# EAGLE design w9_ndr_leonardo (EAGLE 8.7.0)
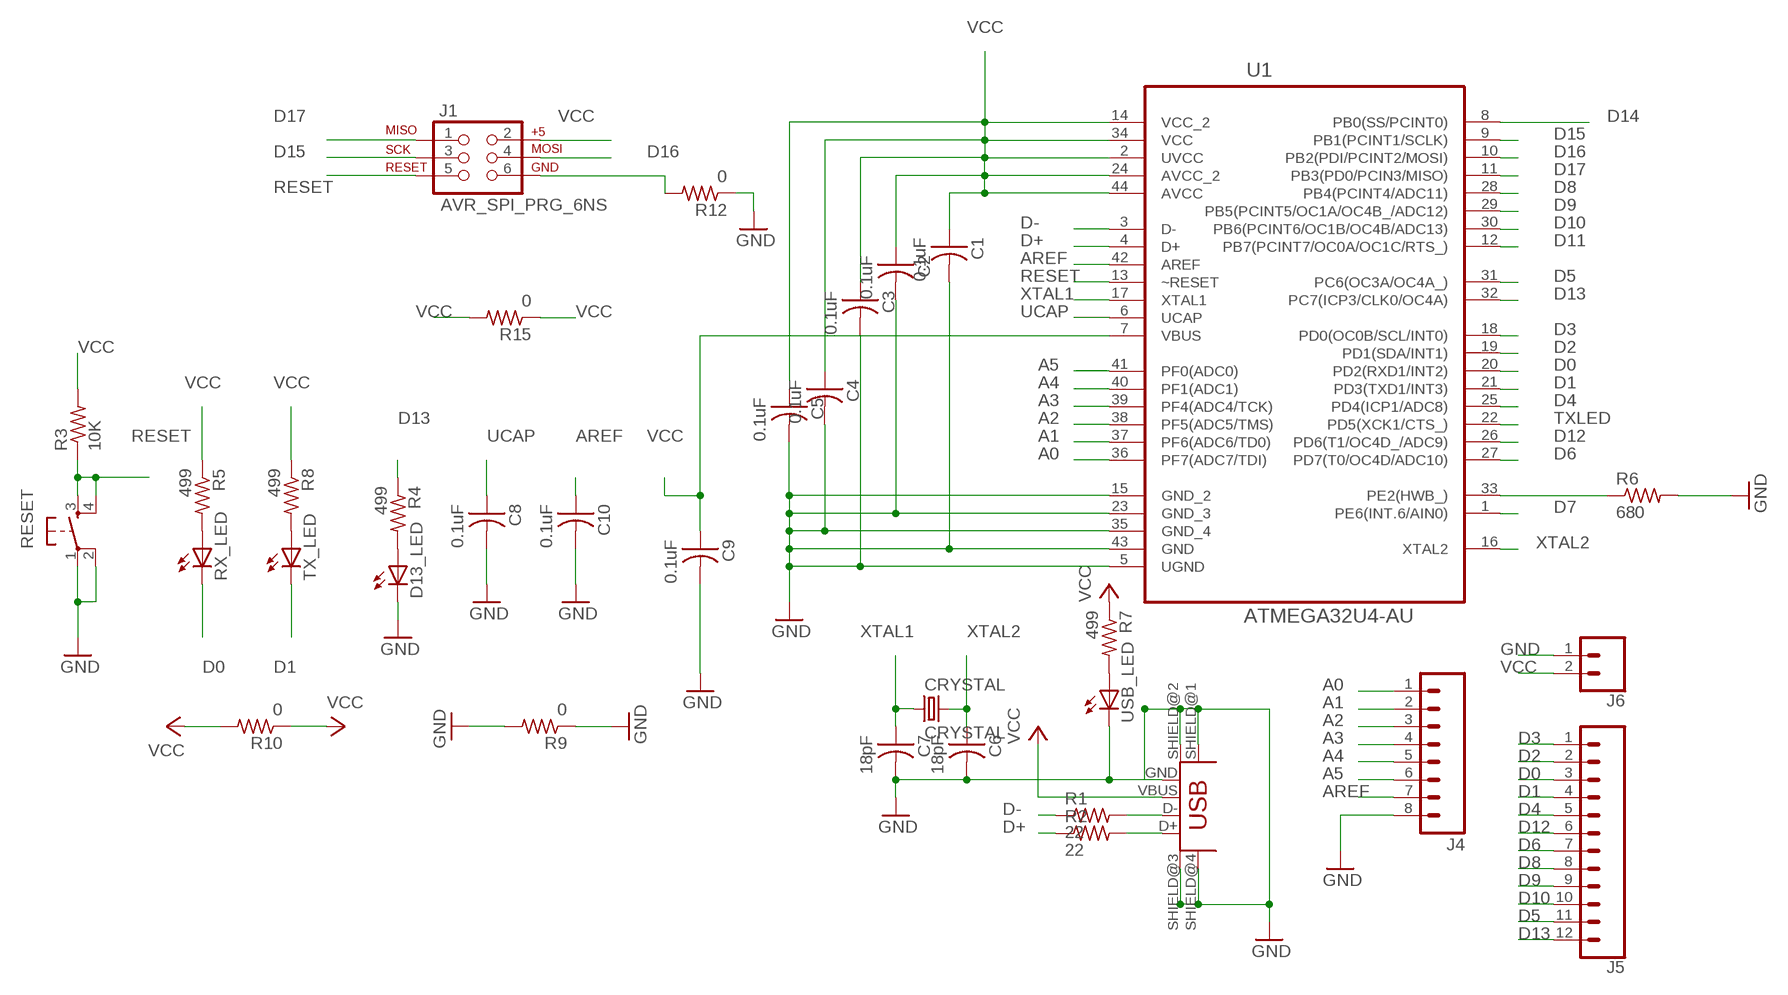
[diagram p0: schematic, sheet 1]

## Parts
C1  0.1uF  CAP-US1206FAB  [C1206FAB]
C2  0.1uF  CAP-US1206FAB  [C1206FAB]
C3  0.1uF  CAP-US1206FAB  [C1206FAB]
C4  0.1uF  CAP-US1206FAB  [C1206FAB]
C5  0.1uF  CAP-US1206FAB  [C1206FAB]
C6  18pF  CAP-US1206FAB  [C1206FAB]
C7  18pF  CAP-US1206FAB  [C1206FAB]
C8  0.1uF  CAP-US1206FAB  [C1206FAB]
C9  0.1uF  CAP-US1206FAB  [C1206FAB]
C10  0.1uF  CAP-US1206FAB  [C1206FAB]
CRYSTAL  CRYSTAL  [2-SMD-5X3MM]
D13_LED  LED1206  [1206]
J1  AVR_SPI_PRG_6NS  [2X3-NS]
J4  M08NO_SILK  [1X08_PIN1_NO_SILK]
J5  CONN_12NO_SILK  [1X12_NO_SILK]
J6  CONN_021X02_NO_SILK  [1X02_NO_SILK]
R1  22  RES-US1206FAB  [R1206FAB]
R2  22  RES-US1206FAB  [R1206FAB]
R3  10K  RES-US1206FAB  [R1206FAB]
R4  499  RESISTOR1206  [1206]
R5  499  RESISTOR1206  [1206]
R6  680  RES-US1206FAB  [R1206FAB]
R7  499  RESISTOR1206  [1206]
R8  499  RESISTOR1206  [1206]
R9  0  RES-US1206FAB  [R1206FAB]
R10  0  RES-US1206FAB  [R1206FAB]
R12  0  RES-US1206FAB  [R1206FAB]
R15  0  RES-US1206FAB  [R1206FAB]
RESET  6MM_SWITCH6MM_SWITCH  [6MM_SWITCH]
RX_LED  LED1206  [1206]
TX_LED  LED1206  [1206]
U1  ATMEGA32U4-AU  [QFP80P1200X1200X120-44N]
USB_LED  LED1206  [1206]
USB_UPLOAD  USB_MINIB  [USB_MINIB]

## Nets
A0: J4.1 U1.36(PF7(ADC7/TDI))
A1: J4.2 U1.37(PF6(ADC6/TD0))
A2: J4.3 U1.38(PF5(ADC5/TMS))
A3: J4.4 U1.39(PF4(ADC4/TCK))
A4: J4.5 U1.40(PF1(ADC1))
A5: J4.6 U1.41(PF0(ADC0))
AREF: C10.1 J4.7 U1.42(AREF)
D0: J5.3 RX_LED.2(C) U1.20(PD2(RXD1/INT2))
D1: J5.4 TX_LED.2(C) U1.21(PD3(TXD1/INT3))
D2: J5.2 U1.19(PD1(SDA/INT1))
D3: J5.1 U1.18(PD0(OC0B/SCL/INT0))
D4: J5.5 U1.25(PD4(ICP1/ADC8))
D5: J5.11 U1.31(PC6(OC3A/OC4A_))
D6: J5.7 U1.27(PD7(T0/OC4D/ADC10))
D7: U1.1(PE6(INT.6/AIN0))
D8: J5.8 U1.28(PB4(PCINT4/ADC11))
D9: J5.9 U1.29(PB5(PCINT5/OC1A/OC4B_/ADC12))
D10: J5.10 U1.30(PB6(PCINT6/OC1B/OC4B/ADC13))
D11: U1.12(PB7(PCINT7/OC0A/OC1C/RTS_))
D12: J5.6 U1.26(PD6(T1/OC4D_/ADC9))
D13: J5.12 R4.1 U1.32(PC7(ICP3/CLK0/OC4A))
D14: U1.8(PB0(SS/PCINT0))
D15: J1.3 U1.9(PB1(PCINT1/SCLK))
D16: J1.4 U1.10(PB2(PDI/PCINT2/MOSI))
D17: J1.1 U1.11(PB3(PD0/PCIN3/MISO))
D+: R2.1 U1.4(D+)
D-: R1.1 U1.3(D-)
GND: C1.2 C2.2 C3.2 C4.2 C5.2 C6.2 C7.2 C8.2 C9.2 C10.2 D13_LED.2(C) J4.8 J6.1 R6.2 R9.1 R9.2 R12.1 RESET.1(P) RESET.2(P1) U1.5(UGND) U1.15(GND_2) U1.23(GND_3) U1.35(GND_4) U1.43(GND) USB_LED.2(C) USB_UPLOAD.GND USB_UPLOAD.SHIELD@1(SHIELD) USB_UPLOAD.SHIELD@2(SHIELD1) USB_UPLOAD.SHIELD@3(SHIELD2) USB_UPLOAD.SHIELD@4(SHIELD3)
N$1: R1.2 USB_UPLOAD.D-
N$2: R2.2 USB_UPLOAD.D+
N$3: D13_LED.1(A) R4.2
N$4: R5.2 RX_LED.1(A)
N$5: R7.2 USB_LED.1(A)
N$6: R8.2 TX_LED.1(A)
N$13: J1.6 R12.2
N$35: R6.1 U1.33(PE2(HWB_))
RESET: J1.5 R3.1 RESET.3(S) RESET.4(S1) U1.13(~RESET)
TXLED: U1.22(PD5(XCK1/CTS_))
UCAP: C8.1 U1.6(UCAP)
VCC: C1.1 C2.1 C3.1 C4.1 C5.1 C9.1 J1.2 J6.2 R3.2 R5.1 R7.1 R8.1 R10.1 R10.2 R15.1 R15.2 U1.2(UVCC) U1.7(VBUS) U1.14(VCC_2) U1.24(AVCC_2) U1.34(VCC) U1.44(AVCC) USB_UPLOAD.VBUS
XTAL1: C7.1 CRYSTAL.P$1 U1.17(XTAL1)
XTAL2: C6.1 CRYSTAL.P$2 U1.16(XTAL2)

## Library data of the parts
C1-C10 = fab:CAP-US
CRYSTAL = fab:CRYSTAL
D13_LED RX_LED TX_LED USB_LED = ng:LED
J1 = SparkFun-ConnectorsModified:AVR_SPI_PRG_6: AVR ISP 6 Pin This is the reduced ISP connector for AVR programming. Common on Arduino. This footprint will take up less PCB space and can be used with a 10-pin to 6-pin adapter such as SKU: BOB-08508 **Special note about "TEST_POINT" package. The stop mask is on the top side, so if you want your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
J4 = SparkFun-ConnectorsModified:M08: Header 8 Standard 8-pin 0.1" header. Use with straight break away headers (SKU : PRT-00116), right angle break away headers (PRT-00553), swiss pins (PRT-00743), machine pins (PRT-00117), and female headers (PRT-00115).
J5 = SparkFun-Connectors:CONN_12: Multi connection point. Often used as Generic Header-pin footprint for 0.1 inch spaced/style header connections On any of the 0.1 inch spaced packages, you can populate with these: Break Away Headers - Straight (PRT-00116) Break Away Male Headers - Right Angle (PRT-00553) Female Headers (PRT-00115)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
J6 = SparkFun-Connectors:CONN_02: Multi connection point. Often used as Generic Header-pin footprint for 0.1 inch spaced/style header connections
R1-R3 R6 R9 R10 R12 R15 = fab:RES-US: Resistor (US Symbol)
R4 R5 R7 R8 = ng:RESISTOR
RESET = fab:6MM_SWITCH: OMRON SWITCH
U1 = Atmel_By_element14_Batch_1:ATMEGA32U4-AU: 8-bit Microcontroller with ISP Flash and USB Controller; MPN: ATMEGA32U4-AU; OC_FARNELL: 1748525; OC_NEWARK: 26R5633; PACKAGE: TQFP-44; SUPPLIER: Atmel
USB_UPLOAD = fab:USB_MINIB

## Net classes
0 default: width 0.305 mm, drill 0.305 mm, clearance 0.305 mm

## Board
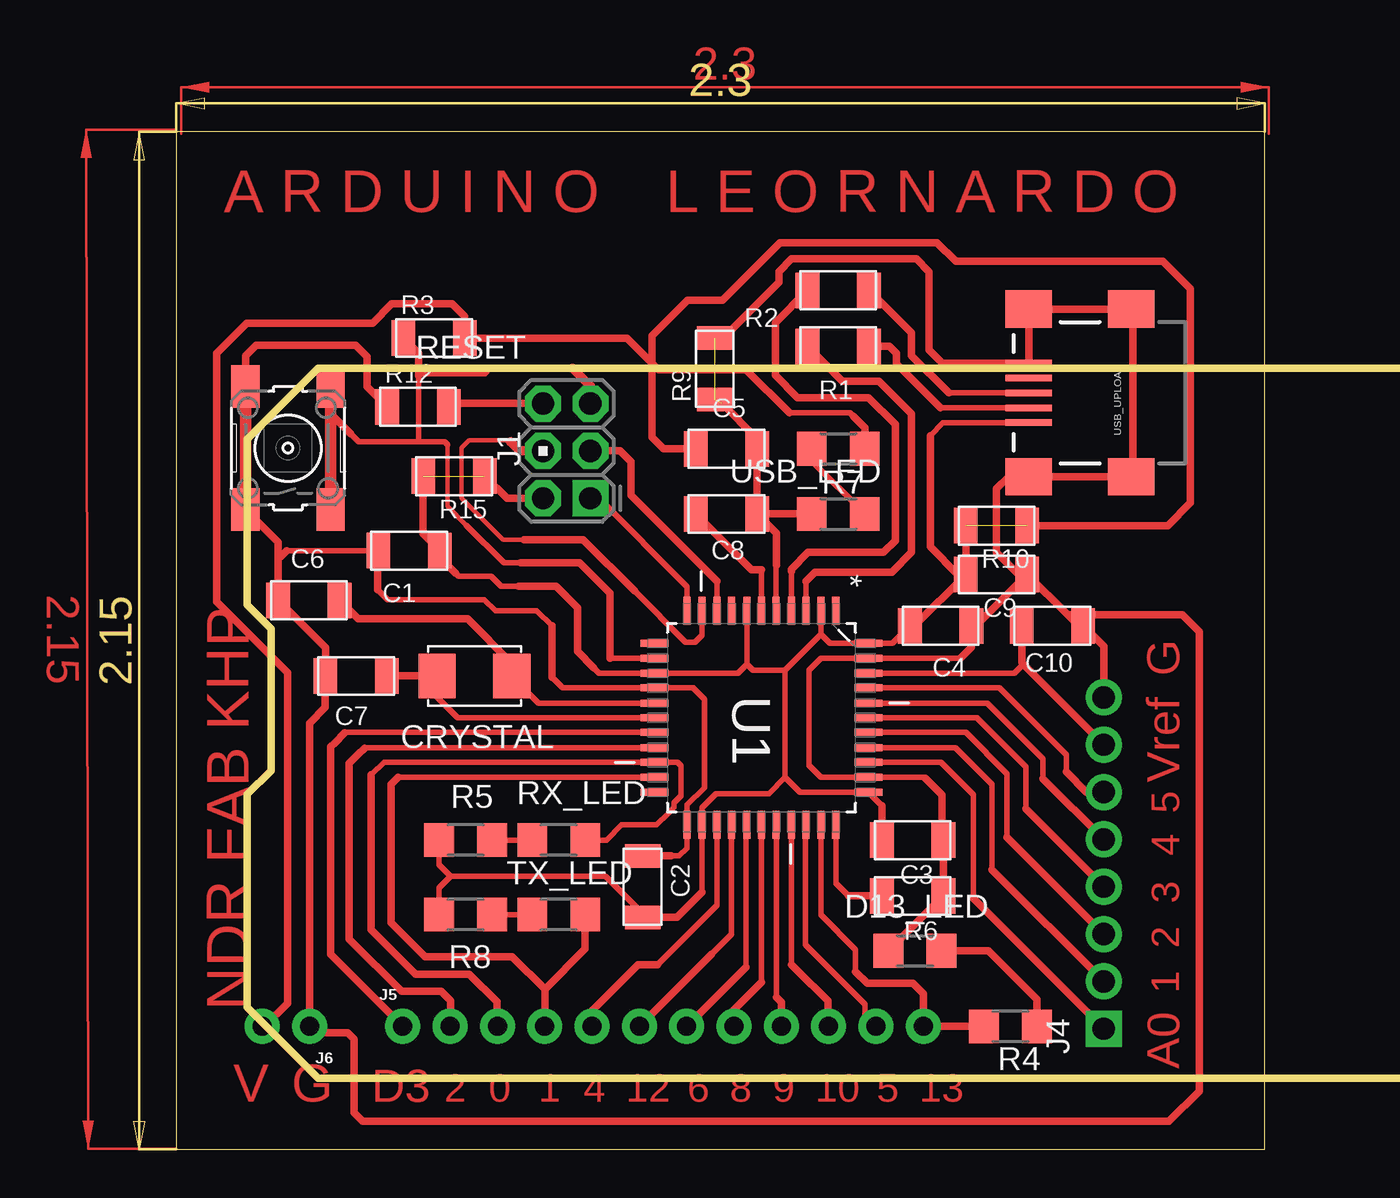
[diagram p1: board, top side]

Size 60.72 x 56.42 mm. Coordinates in mm from the lower left corner, seen from the top.
Outline: 2.3,0 60.72,0 60.72,54.61 2.3,54.61 2.3,0
Copper layers (1*16): Top 0.035mm / dielectric 1.5mm / Bottom 0.035mm
Design rules "default *": minimum track width 10mil, minimum drill 24mil, track to track 0.4mm, track to pad 0.4mm, pad to pad 0.4mm, via to via 0.4mm, smd to smd 0.4mm, copper to edge 40mil, drill to drill 0.4mm, minimum pad ring 10mil, minimum via ring 8mil, stop-mask expansion 4mil, vias tented up to drill 0mil, thermal gap 10mil
Milling: area 6.1,3.8 to 106.4,41.9

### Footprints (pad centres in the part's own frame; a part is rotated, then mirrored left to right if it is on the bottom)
C1206FAB = smd 1.27 x 1.905: 1 -1.651,0; 2 1.651,0
2-SMD-5X3MM = smd 2 x 2.4: P$1 -2,0; P$2 2,0
1206 = smd 1.6 x 1.803: 1 -1.422,0; 2 1.422,0
2X3-NS = drill 1.2 pad 1.93 square: 1 -2.54,-1.27 | drill 1.2 pad 1.93 octagon: 2 -2.54,1.27; 3 0,-1.27; 4 0,1.27; 5 2.54,-1.27; 6 2.54,1.27
1X08_PIN1_NO_SILK = drill 1.2 pad 1.93 square: 1 0,0 | drill 1.2 pad 1.93: 2 2.54,0; 3 5.08,0; 4 7.62,0; 5 10.16,0; 6 12.7,0; 7 15.24,0; 8 17.78,0
1X12_NO_SILK = drill 1.016 pad 1.88: 1 0,0; 2 2.54,0; 3 5.08,0; 4 7.62,0; 5 10.16,0; 6 12.7,0; 7 15.24,0; 8 17.78,0; 9 20.32,0; 10 22.86,0; 11 25.4,0; 12 27.94,0
1X02_NO_SILK = drill 1.016 pad 1.88: 1 0,0; 2 2.54,0
R1206FAB = smd 1.27 x 1.905: 1 -1.651,0; 2 1.651,0
6MM_SWITCH = smd 2.286 x 1.524: 1 -3.302,2.286; 2 3.302,2.286; 3 -3.302,-2.286; 4 3.302,-2.286
QFP80P1200X1200X120-44N = smd 1.5 x 0.38: 1 -5.74,3.988; 2 -5.74,3.2; 3 -5.74,2.388; 4 -5.74,1.6; 5 -5.74,0.787; 6 -5.74,0; 7 -5.74,-0.787; 8 -5.74,-1.6; 9 -5.74,-2.388; 10 -5.74,-3.2; 11 -5.74,-3.988; 23 5.74,-3.988; 24 5.74,-3.2; 25 5.74,-2.388; 26 5.74,-1.6; 27 5.74,-0.787; 28 5.74,0; 29 5.74,0.787; 30 5.74,1.6; 31 5.74,2.388; 32 5.74,3.2; 33 5.74,3.988 | smd 0.38 x 1.5: 12 -3.988,-5.74; 13 -3.2,-5.74; 14 -2.388,-5.74; 15 -1.6,-5.74; 16 -0.787,-5.74; 17 0,-5.74; 18 0.787,-5.74; 19 1.6,-5.74; 20 2.388,-5.74; 21 3.2,-5.74; 22 3.988,-5.74; 34 3.988,5.74; 35 3.2,5.74; 36 2.388,5.74; 37 1.6,5.74; 38 0.787,5.74; 39 0,5.74; 40 -0.787,5.74; 41 -1.6,5.74; 42 -2.388,5.74; 43 -3.2,5.74; 44 -3.988,5.74
USB_MINIB = smd 2.5 x 0.35: D+ 3.77,0; D- 3.77,0.8; GND 3.77,-1.6; ID 3.77,-0.8; VBUS 3.77,1.6 | smd 2.5 x 2: SHIELD@1 -1.73,-4.5; SHIELD@2 -1.73,4.5; SHIELD@3 3.77,4.5; SHIELD@4 3.77,-4.5

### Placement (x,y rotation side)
C1  14.8,32.13 180 top
C2  27.33,14.09 90 top
C3  41.83,16.59 0 top
C4  43.33,28.09 0 top
C5  31.83,37.59 0 top
C6  9.41,29.46 180 top
C7  11.95,25.4 180 top
C8  31.83,34.09 0 top
C9  46.33,30.84 0 top
C10  49.33,28.09 0 top
CRYSTAL  18.3,25.4 0 top
D13_LED  41.96,10.66 180 top
J1  23.26,37.48 90 top
J4  52.08,6.47 90 top
J5  14.46,6.59 0 top
J6  9.46,6.59 180 top
R1  37.83,43.09 0 top
R2  37.83,46.09 0 top
R3  16.13,43.54 0 top
R4  47.08,6.59 0 top
R5  17.83,16.59 0 top
R6  41.83,13.59 0 top
R7  37.83,37.59 180 top
R8  17.83,12.59 0 top
R9  31.2,41.88 90 top
R10  46.33,33.47 180 top
R12  15.27,39.84 0 top
R15  17.21,36.12 180 top
RESET  8.29,37.63 90 top
RX_LED  22.83,16.59 0 top
TX_LED  22.83,12.59 0 top
U1  33.71,23.16 270 top
USB_LED  37.83,34.09 180 top
USB_UPLOAD  51.83,40.59 180 top

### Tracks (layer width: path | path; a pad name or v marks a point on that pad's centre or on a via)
A0
  Top 0.305: U1.36 43.34,20.77 45.08,19.03 45.08,13.47
  Top 0.406: 45.08,13.47 J4.1
A1
  Top 0.305: U1.37 44.12,21.56 46.08,19.59 46.08,15.01
  Top 0.406: 46.08,15.01 J4.2
A2
  Top 0.305: U1.38 44.68,22.37 46.89,20.16 46.89,16.74
  Top 0.406: 46.89,16.74 J4.3
A3
  Top 0.305: U1.39 45.27,23.16 47.89,20.53 47.89,18.28
  Top 0.406: 47.89,18.28 J4.4
A4
  Top 0.305: U1.40 45.85,23.95 48.83,20.97 48.83,19.88
  Top 0.406: 48.83,19.88 J4.5
A5
  Top 0.305: U1.41 46.49,24.76 50.08,21.17 50.08,20.25
  Top 0.406: 50.08,20.25 51.16,19.17 J4.6
AREF
  Top 0.305: U1.42 47.28,25.55 47.76,26.03
  Top 0.406: J4.7 47.76,26.03 47.68,26.11 C10.1
D0
  Top 0.305: 12.77,20.09 13.46,20.78 U1.20 27.98,20.78 29.21,20.78 29.39,20.59 29.39,20.34 29.39,18.97 29.02,18.59 29.02,18.34 28.69,18.02 28.08,17.41 26.21,17.41 25.39,16.59 RX_LED.2
  Top 0.406: 12.77,20.09 12.77,11.78 15.14,9.41 18.02,9.41 19.52,7.91 19.52,6.61 J5.3 19.58,6.59
D1
  Top 0.305: 14.21,19.97 14.22,19.96 U1.21
  Top 0.406: 14.21,19.97 13.83,19.59 13.83,12.16 15.64,10.34 20.33,10.34 22.08,8.59 | 22.08,8.59 J5.4 | TX_LED.2 24.25,10.77 22.08,8.59
D2
  Top 0.305: U1.19 12.42,21.56 12.05,21.19
  Top 0.406: 12.39,21.53 12.05,21.19 11.58,20.72 11.58,11.28 14.39,8.47 16.52,8.47 17.02,7.97 17.02,6.62 J5.2
D3
  Top 0.305: 10.82,21.83 11.36,22.37 U1.18
  Top 0.406: 11.33,22.34 10.82,21.83 10.58,21.59 10.58,10.47 J5.1
D4
  Top 0.305: U1.25 31.33,13.09 28.14,9.91
  Top 0.406: J5.5 24.62,7.44 27.08,9.91 28.14,9.91
D5
  Top 0.305: U1.31 36.08,17.4 36.08,10.97 39.27,7.78 39.27,7.18 J5.11
D6
  Top 0.305: U1.27 32.89,17.39 32.89,9.78
  Top 0.406: J5.7 32.32,9.2 32.89,9.78
D8
  Top 0.305: 33.71,8.97 U1.28
  Top 0.406: 33.71,8.97 32.21,7.47 32.21,6.62 J5.8
D9
  Top 0.305: U1.29 34.52,17.4 34.52,8.16
  Top 0.406: J5.9 34.78,7.9 34.66,8.02 34.52,8.16
D10
  Top 0.305: 35.6,9.64 35.31,9.93 U1.30
  Top 0.406: 35.33,9.91 35.6,9.64 37.27,7.97 37.27,6.64 J5.10
D12
  Top 0.305: U1.26 32.11,11.55 31.03,10.46
  Top 0.406: J5.6 31.03,10.46
D13
  Top 0.305: 38.77,9.53 38.77,10.72 36.91,12.58 U1.32
  Top 0.406: R4.1 J5.12 42.39,8.34 41.83,8.91 39.39,8.91 38.77,9.53
D15
  Top 0.305: U1.9 31.32,30.48
  Top 0.406: J1.3 26.13,37.48 26.71,36.91 26.71,35.09 31.32,30.48
D16
  Top 0.254: 20.96,32.72 19.83,32.72 17.61,34.94 17.61,37.66 18.02,38.06 20.14,38.06 20.24,37.97 20.36,37.84
  Top 0.305: U1.10 30.51,27.59 30.14,27.22 29.64,27.22 26.89,29.97
  Top 0.406: 26.89,29.97 24.14,32.72 20.96,32.72
  Top 0.508: J1.4 20.73,37.48 20.24,37.97
D17
  Top 0.305: U1.11 29.72,30.2 24.98,34.94 J1.1
D+
  Top 0.305: U1.4 35.31,31.01
  Top 0.406: 35.31,31.01 35.31,31.14 36.21,32.03 40.27,32.03 40.89,32.66 40.89,38.91 39.46,40.34 35.64,40.34 34.46,41.53 34.46,44.37 R2.1
D-
  Top 0.305: U1.3 36.1,30.49
  Top 0.406: R1.1 38.05,41.22 40.02,41.22 41.77,39.47 41.77,32.03 40.71,30.97 36.58,30.97 36.1,30.49
GND  (2 unrouted)
  Top 0.305: U1.5 34.5,31.32 34.52,31.34 | 22.46,25.34 23.04,24.76 U1.15 30.06,24.76 30.06,24.74 30.64,24.16 30.64,19.41 29.72,18.49 U1.23 29.71,17.4 29.71,16.16 29.3,15.74 28.86,15.74 | RESET.1 6.52,33.82 | 44.39,26.36 U1.43 36.91,26.36 36.25,25.7 36.25,20.62 36.91,19.96 U1.35 42.47,19.96 42.52,19.91 | C1.2 8.21,32.13 | 22.46,28.09 21.64,28.91 19.43,28.91 18.83,29.5 13.64,29.5 13.11,30.03
  Top 0.406: 42.52,19.91 43.39,19.03 43.39,16.68 C3.2 R6.2 D13_LED.2 | 53.39,36.09 USB_UPLOAD.SHIELD@3 46.99,36.09 46.33,35.44 46.33,32.03 47.75,30.61 | 53.39,36.09 USB_UPLOAD.SHIELD@2 | RESET.2 6.01,42.59 6.57,43.16 11.93,43.16 12.55,42.53 12.55,40.91 R12.1 | C2.2 28.86,15.74 | 34.52,31.34 34.52,33.06 C8.2 | C8.2 USB_LED.2 | C8.2 C5.2 33.48,38.13 31.58,40.03 | 22.46,25.34 22.46,28.09 | J4.8 52.08,27 C10.2 50.73,28.09 50.15,28.68 | 50.15,28.68 C9.2 47.75,30.61 | 47.75,30.61 45.23,28.09 C4.2 44.98,26.95 44.39,26.36 | 9.52,6.53 J6.1 | 53.39,36.09 53.64,36.34 53.64,45.01 USB_UPLOAD.SHIELD@1 USB_UPLOAD.SHIELD@4 USB_UPLOAD.GND 43.42,42.19 42.71,42.91 42.71,47.09 42.02,47.78 35.33,47.78 34.64,47.09 34.64,46.53 31.65,43.53 R9.2 | 13.11,30.03 13.11,32.09 C1.2 | J6.1 9.8,6.25 11.49,6.25 11.85,5.89 11.85,1.95 12.3,1.5 55.58,1.5 57.21,3.12 57.21,27.77 56.3,28.68 50.15,28.68 | 7.76,31.81 C6.2 10.3,26.92 C7.2 10.3,23.72 9.46,22.88 J6.1 | 7.76,31.81 7.76,32.58 6.52,33.82 | 8.21,32.13 7.9,31.81 7.76,31.81
  Top 0.61: RESET.1 RESET.2
N$1
  Top 0.305: USB_UPLOAD.D- 43.32,39.79
  Top 0.406: 43.32,39.79 40.96,42.16 40.96,42.72 40.58,43.09 R1.2
N$2
  Top 0.305: USB_UPLOAD.D+ 43.77,40.59
  Top 0.406: 43.77,40.59 41.77,42.59 41.77,43.81 R2.2
N$3
  Top 0.406: R4.2 48.5,8.05 45.89,10.66 D13_LED.1
N$4
  Top 0.305: R5.2 RX_LED.1
N$5
  Top 0.305: R7.2 36.41,36.94 USB_LED.1
N$6
  Top 0.305: R8.2 TX_LED.1
N$13
  Top 0.406: R12.2 17.11,40.03 21.98,40.03
  Top 0.508: 21.98,40.03 J1.6
N$35
  Top 0.305: U1.33 37.7,14.88 37.7,14.48 37.7,14.29 38.39,13.59
  Top 0.406: 38.39,13.59 R6.1
RESET
  Top 0.254: 17.86,33.5 16.86,34.5 16.86,37.81
  Top 0.305: U1.13 25.6,26.36 25.58,26.34 | 20.77,31.47 19.89,31.47 17.86,33.5 | 16.86,37.81 16.71,37.97 15.3,37.97 | 15.3,37.97 12.08,37.97 11.64,38.41 | 15.3,41.5 15.3,37.97 | 19.14,41.91 18.86,41.62 15.36,41.62 15.3,41.69
  Top 0.406: RESET.4 10.58,39.47 11.64,38.41 | 25.58,26.34 25.58,29.84 23.96,31.47 20.77,31.47 | 23.58,41.91 19.14,41.91 | R3.1 15.3,42.72 15.3,41.69 15.3,41.5
  Top 0.508: J1.5 24.53,40.96 23.58,41.91
  Top 0.61: RESET.4 RESET.3
UCAP
  Top 0.305: U1.6 33.71,31.09
  Top 0.406: 33.71,31.09 33.18,31.09 C8.1
VCC  (2 unrouted)
  Top 0.305: 34.98,19.97 34.98,25.7 | U1.7 32.92,26.03 | 36.91,27.63 37.39,27.15 U1.44 40.73,27.15 C4.1 | 36.91,27.63 34.98,25.7 | 32.92,26.03 32.44,25.55 U1.14 25,25.55 24.71,25.84 | 34.98,25.7 33.26,25.7 32.92,26.03 | 34.98,19.97 35.78,19.17 U1.34 40.18,18.44 | 34.98,19.97 34.11,19.09 31.27,19.09 30.51,18.34 U1.24 30.52,13.78 | 36.91,27.63 U1.2 | C2.1 27.33,12.66 25.33,14.66 17.02,14.66 | R5.1 16.41,15.27 17.02,14.66 | R8.1 16.41,14.05 17.02,14.66 | 38.64,39.34 38.46,39.53 35.21,39.53 | USB_UPLOAD.VBUS 43.46,38.99 42.77,38.31 | 17.3,30.91 17.46,30.75 19.21,30.75 19.74,30.22 20.68,30.22 20.83,30.22
  Top 0.406: C2.1 29.18,12.44 30.52,13.78 | C5.1 28.46,37.59 27.83,38.22 27.83,42.19 | R7.1 39.25,38.73 38.64,39.34 | 35.21,39.53 32.89,41.84 28.18,41.84 27.83,42.19 | C4.1 41.93,28.09 C9.1 | 44.6,30.92 C9.1 | C9.1 44.83,31 44.68,31.15 R10.2 | J6.2 7.02,6.59 8.27,7.84 8.27,25.56 4.46,29.38 4.46,42.72 6.08,44.34 12.83,44.34 13.86,45.38 17.11,45.38 17.78,44.7 R3.2 26.48,43.54 27.83,42.19 | C9.1 44.27,30.84 42.77,32.34 42.77,38.31 | C3.1 40.18,18.44 | C1.1 | 17.3,30.91 16.45,31.75 C1.1 | R15.1 20.04,34.94 J1.2 | R15.2 15.55,33.02 C1.1 | 27.83,42.19 27.83,43.66 29.74,45.56 31.61,45.56 34.71,48.66 43.14,48.66 44.14,47.66 55.27,47.66 56.74,46.19 56.74,34.69 55.52,33.47 R10.1 | 24.71,25.84 23.83,26.72 23.83,29.06 22.68,30.22 20.68,30.22
XTAL1
  Top 0.305: U1.17 17.39,23.16 16.3,24.25 CRYSTAL.P$1
  Top 0.406: C7.1 CRYSTAL.P$1
XTAL2
  Top 0.305: CRYSTAL.P$2 21.76,23.95 U1.16
  Top 0.406: C6.1 12.06,28.47 17.93,28.47 20.3,26.09 CRYSTAL.P$2
(copper drawn outside any net)
  shapes: Top area x2

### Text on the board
Top: A R D U I N O L E O R N A R D O | G | Vref | 5 | 4 | 3 | 2 | 1 | NDR FAB KHP | A0 | V | G | D3 | 2 | 0 | 1 | 4 | 12 | 6 | 8 | 9 | 10 | 5 | 13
